|   IBIS model for TI AM261
[IBIS Ver]   5.1
[Disclaimer]   Please be aware that in the absence of a written agreement
|   Texas Instruments(TI) assumes no liability for:
|   (1) The accuracy of the IBIS models provided to your company,
|   however, the IBIS model is compliant to industry standard
|   IQ Level 2a.  Refer to IBIS Quality Section below for
|   for full details.
|   (2) The proper functioning of these Models in your design
|   or for any resulting applications
|   (3) Infringement of patents, copyrights or intellectual
|   property rights resulting from your use of these
|   models.
|   TI provides IBIS Models as a service to our customers and
|   therefore reserves the right to limit distribution of the
|   Models.  The information is subject to change without notice.
[File Name]  zcz.ibs
[File Rev]   0.1
|   -Initial version
|   -Updated Package model
[Date]   10 October 2024
[Source]   Texas Instruments Incorporated
[Copyright]   Property of Texas Instruments Incorporated.
|   Unauthorized reproduction and/or distribution is strictly.
|   prohibited.
|   This product is protected under copyright law and trade
|   secret law as an unpublished work.
|   Created 2012,(C) Copyright 1999-2012,
|   Texas Instruments Incorporated., All Rights Reserved.
|   These commodities are under the U.S. Government
|   distribution license control. As such,they are not to be
|   re-exported without the prior approval of the U.S.
|   Department of Commerce.
[Notes]
   ADC pins are marked as NC
   USB pins are marked as NC
   Clock pins are marked as NC
   nReset pin marked as NC
|   Revision History
|   GERNERAL COMMENT: All IBIS Quality Notes below reflect latest release
|   and version of IBIS File
|   File passes ibischk6.0 with 0 errors and 35 warnings
|   Component AM261
[Component] AM261
[Manufacturer] TEXAS INSTRUMENTS
[Package Model] AM261_ZCZ
[Package]
|   typ   min   max
R_pkg   0.22926   0.10115   0.40448
L_pkg   4.031e-9   1.747e-9   8.28e-9
C_pkg   5.339e-13   3.606e-13   8.638e-13
[Pin]   Signal_name   model_name
E9   VDD   POWER
E11   VDD   POWER
F9   VDD   POWER
F11   VDD   POWER
G5   VDD   POWER
G6   VDD   POWER
G13   VDD   POWER
G14   VDD   POWER
K5   VDD   POWER
K6   VDD   POWER
K13   VDD   POWER
K14   VDD   POWER
N5   VDD   POWER
N6   VDD   POWER
N13   VDD   POWER
N14   VDD   POWER
R6   VDDA18_LDO   POWER
R8   VDDA18_LDO   POWER
R11   VDDA18_LDO   POWER
R4   VDDA18_OSC_PLL   POWER
P7   VDDA33   POWER
P9   VDDA33   POWER
P11   VDDA33   POWER
D10   VDDAR2   POWER
H3   VDDAR3   POWER
D6   VDDS18   POWER
E15   VDDS18   POWER
L4   VDDS18   POWER
N15   VDDS18   POWER
T3   VDDS18_LDO   POWER
D8   VDDS33   POWER
D12   VDDS33   POWER
H4   VDDS33   POWER
H15   VDDS33   POWER
L15   VDDS33   POWER
P4   VDDS33   POWER
R15   VDDS33   POWER
T4   VDD_TEMP   NC
J16   VNWA   POWER
N3   VPP   POWER
V15   ADC0_AIN0   NC
U15   ADC0_AIN1   NC
T14   ADC0_AIN2   NC
U14   ADC0_AIN3   NC
U13   ADC0_AIN4   NC
R14   ADC0_AIN5   NC
T11   ADC1_AIN0   NC
U11   ADC1_AIN1   NC
T12   ADC1_AIN2   NC
V12   ADC1_AIN3   NC
U12   ADC1_AIN4   NC
R12   ADC1_AIN5   NC
R10   ADC2_AIN0   NC
T10   ADC2_AIN1   NC
U10   ADC2_AIN2   NC
T9   ADC2_AIN3   NC
V9   ADC2_AIN4   NC
T8   ADC2_AIN5   NC
U16   ADC_CAL0   NC
V14   ADC_VREFHI_G0   NC
V10   ADC_VREFHI_G1   NC
V13   ADC_VREFLO_G0   NC
V11   ADC_VREFLO_G1   NC
T6   ATESTV1   NC
M2   CLKOUT0   bc1833dv40dcpbfbp18ll_rxll_ssdlv
T5   DAC_OUT   NC
T13   DAC_VREF0   NC
B2   EPWM0_A   bc1833dv40dcpbfbp18ll_rxll_ssdlh_135u
B1   EPWM0_B   bc1833dv40dcpbfbp18ll_rxll_ssdlh_135u
D3   EPWM1_A   bc1833dv40dcpbfbp18ll_rxll_ssdlh_135u
D2   EPWM1_B   bc1833dv40dcpbfbp18ll_rxll_ssdlh_135u
C2   EPWM2_A   bc1833dv40dcpbfbp18ll_rxll_ssdlh_135u
C1   EPWM2_B   bc1833dv40dcpbfbp18ll_rxll_ssdlh_135u
E2   EPWM3_A   bc1833dv40dcpbfbp18ll_rxll_ssdlh_135u
E3   EPWM3_B   bc1833dv40dcpbfbp18ll_rxll_ssdlv
D1   EPWM4_A   bc1833dv40dcpbfbp18ll_rxll_ssdlv
E4   EPWM4_B   bc1833dv40dcpbfbp18ll_rxll_ssdlv
F2   EPWM5_A   bc1833dv40dcpbfbp18ll_rxll_ssdlv
G2   EPWM5_B   bc1833dv40dcpbfbp18ll_rxll_ssdlv
E1   EPWM6_A   bc1833dv40dcpbfbp18ll_rxll_ssdlv
F3   EPWM6_B   bc1833dv40dcpbfbp18ll_rxll_ssdlv
F4   EPWM7_A   bc1833dv40dcpbfbp18ll_rxll_ssdlv
F1   EPWM7_B   bc1833dv40dcpbfbp18ll_rxll_ssdlv
G3   EPWM8_A   bc1833dv40dcpbfbp18ll_rxll_ssdlv
H2   EPWM8_B   bc1833dv40dcpbfbp18ll_rxll_ssdlv
G1   EPWM9_A   bc1833dv40dcpbfbp18ll_rxll_ssdlv
J2   EPWM9_B   bc1833dv40dcpbfbp18ll_rxll_ssdlv
B14   EQEP0_A   bc1833dv40dcpbfbp18ll_rxll_ssdlh
A14   EQEP0_B   bc1833dv40dcpbfbp18ll_rxll_ssdlh
D11   EQEP0_INDEX   bc1833dv40dcpbfbp18ll_rxll_ssdlh
C12   EQEP0_STROBE   bc1833dv40dcpbfbp18ll_rxll_ssdlh
P2   EXT_REFCLK0   bc1833dv40dcpbfbp18ll_rxll_ssdlh
G4   GPIO63   bc1833dv40dcpbfbp18ll_rxll_ssdlv
J3   GPIO64   bc1833dv40dcpbfbp18ll_rxll_ssdlv
H1   GPIO65   bc1833dv40dcpbfbp18ll_rxll_ssdlv
J1   GPIO66   bc1833dv40dcpbfbp18ll_rxll_ssdlv
B12   GPIO136   bc1833dv40dcpbfbp18ll_rxll_ssdlv
A12   GPIO137   bc1833dv40dcpbfbp18ll_rxll_ssdlv
A13   I2C0_SCL   bi2c1833dvfzp18_ssdlh
B13   I2C0_SDA   bi2c1833dvfzp18_ssdlh
D7   I2C1_SCL   bc1833dv40dcpbfbp18ll_rxll_ssdlh
C8   I2C1_SDA   bc1833dv40dcpbfbp18ll_rxll_ssdlh
A9   LIN1_RXD   bc1833dv40dcpbfbp18ll_rxll_ssdlh
B9   LIN1_TXD   bc1833dv40dcpbfbp18ll_rxll_ssdlh
B8   LIN2_RXD   bc1833dv40dcpbfbp18ll_rxll_ssdlh
A8   LIN2_TXD   bc1833dv40dcpbfbp18ll_rxll_ssdlh
M1   MCAN0_RX   bc1833dv40dcpbfbp18ll_rxll_ssdlv
L1   MCAN0_TX   bc1833dv40dcpbfbp18ll_rxll_ssdlv
L2   MCAN1_RX   bc1833dv40dcpbfbp18ll_rxll_ssdlv
K1   MCAN1_TX   bc1833dv40dcpbfbp18ll_rxll_ssdlv
M17   MDIO0_MDC   bc1833dv40dcpbfbp18ll_rxll_ssdlv_135u
N16   MDIO0_MDIO   bc1833dv40dcpbfbp18ll_rxll_ssdlv_135u
A5   MMC0_CD   bc1833dv40dcpbfbp18ll_rxll_ssdlh_135u
B6   MMC0_CLK   bc1833dv40dcpbfbp18ll_rxll_ssdlh_135u
A4   MMC0_CMD   bc1833dv40dcpbfbp18ll_rxll_ssdlh_135u
B5   MMC0_D0   bc1833dv40dcpbfbp18ll_rxll_ssdlh_135u
B4   MMC0_D1   bc1833dv40dcpbfbp18ll_rxll_ssdlh_135u
A3   MMC0_D2   bc1833dv40dcpbfbp18ll_rxll_ssdlh_135u
A2   MMC0_D3   bc1833dv40dcpbfbp18ll_rxll_ssdlh_135u
C6   MMC0_WP   bc1833dv40dcpbfbp18ll_rxll_ssdlh_135u
R2   PORZ   ihhv1833dvhyp18ll_ssdhv
L18   PR0_MDIO0_MDC   bc1833dv40dcpbfbp18ll_rxll_ssdlv_135u
L17   PR0_MDIO0_MDIO   bc1833dv40dcpbfbp18ll_rxll_ssdlv_135u
K17   PR0_PRU0_GPO0   bc1833dv40dcpbfbp18ll_rxll_ssdlv_135u
K18   PR0_PRU0_GPO1   bc1833dv40dcpbfbp18ll_rxll_ssdlv_135u
J18   PR0_PRU0_GPO2   bc1833dv40dcpbfbp18ll_rxll_ssdlv_135u
J17   PR0_PRU0_GPO3   bc1833dv40dcpbfbp18ll_rxll_ssdlv_135u
K16   PR0_PRU0_GPO4   bc1833dv40dcpbfbp18ll_rxll_ssdlv_135u
G17   PR0_PRU0_GPO5   bc1833dv40dcpbfbp18ll_rxll_ssdlv_135u
K15   PR0_PRU0_GPO6   bc1833dv40dcpbfbp18ll_rxll_ssdlv_135u
G15   PR0_PRU0_GPO8   bc1833dv40dcpbfbp18ll_rxll_ssdlv_135u
F17   PR0_PRU0_GPO9   bc1833dv40dcpbfbp18ll_rxll_ssdlv_135u
G18   PR0_PRU0_GPO10   bc1833dv40dcpbfbp18ll_rxll_ssdlv_135u
M16   PR0_PRU0_GPO11   bc1833dv40dcpbfbp18ll_rxll_ssdlv_135u
M15   PR0_PRU0_GPO12   bc1833dv40dcpbfbp18ll_rxll_ssdlv_135u
H17   PR0_PRU0_GPO13   bc1833dv40dcpbfbp18ll_rxll_ssdlv_135u
H16   PR0_PRU0_GPO14   bc1833dv40dcpbfbp18ll_rxll_ssdlv_135u
L16   PR0_PRU0_GPO15   bc1833dv40dcpbfbp18ll_rxll_ssdlv_135u
H18   PR0_PRU0_GPO16   bc1833dv40dcpbfbp18ll_rxll_ssdlv_135u
F18   PR0_PRU1_GPO0   bc1833dv40dcpbfbp18ll_rxll_ssdlv_135u
G16   PR0_PRU1_GPO1   bc1833dv40dcpbfbp18ll_rxll_ssdlv_135u
E17   PR0_PRU1_GPO2   bc1833dv40dcpbfbp18ll_rxll_ssdlv_135u
E18   PR0_PRU1_GPO3   bc1833dv40dcpbfbp18ll_rxll_ssdlv_135u
F16   PR0_PRU1_GPO4   bc1833dv40dcpbfbp18ll_rxll_ssdlv_135u
F15   PR0_PRU1_GPO5   bc1833dv40dcpbfbp18ll_rxll_ssdlv_135u
E16   PR0_PRU1_GPO6   bc1833dv40dcpbfbp18ll_rxll_ssdlv_135u
D18   PR0_PRU1_GPO8   bc1833dv40dcpbfbp18ll_rxll_ssdlv_135u
C18   PR0_PRU1_GPO9   bc1833dv40dcpbfbp18ll_rxll_ssdlv_135u
D17   PR0_PRU1_GPO10   bc1833dv40dcpbfbp18ll_rxll_ssdlv_135u
B18   PR0_PRU1_GPO11   bc1833dv40dcpbfbp18ll_rxll_ssdlv_135u
B17   PR0_PRU1_GPO12   bc1833dv40dcpbfbp18ll_rxll_ssdlv_135u
D16   PR0_PRU1_GPO13   bc1833dv40dcpbfbp18ll_rxll_ssdlv_135u
C17   PR0_PRU1_GPO14   bc1833dv40dcpbfbp18ll_rxll_ssdlv_135u
A17   PR0_PRU1_GPO15   bc1833dv40dcpbfbp18ll_rxll_ssdlv_135u
C16   PR0_PRU1_GPO16   bc1833dv40dcpbfbp18ll_rxll_ssdlv_135u
C15   PR0_PRU1_GPO18   bc1833dv40dcpbfbp18ll_rxll_ssdlv_135u
D15   PR0_PRU1_GPO19   bc1833dv40dcpbfbp18ll_rxll_ssdlh
K2   PR1_PRU0_GPO0   bc1833dv40dcpbfbp18ll_rxll_ssdlv
J4   PR1_PRU0_GPO1   bc1833dv40dcpbfbp18ll_rxll_ssdlv
K4   PR1_PRU0_GPO2   bc1833dv40dcpbfbp18ll_rxll_ssdlv
K3   PR1_PRU0_GPO9   bc1833dv40dcpbfbp18ll_rxll_ssdlv
V17   PR1_PRU1_GPO0   bc1833dv40dcpbfbp18ll_rxll_ssdlh
T16   PR1_PRU1_GPO1   bc1833dv40dcpbfbp18ll_rxll_ssdlh
P15   PR1_PRU1_GPO2   bc1833dv40dcpbfbp18ll_rxll_ssdlh
R16   PR1_PRU1_GPO9   bc1833dv40dcpbfbp18ll_rxll_ssdlh
N2   QSPI0_CLK   bc1833dv40dcpbfbp18ll_rxll_ssdlv
P1   QSPI0_CSN0   bc1833dv40dcpbfbp18ll_rxll_ssdlv
R3   QSPI0_CSN1   bc1833dv40dcpbfbp18ll_rxll_ssdlv
N1   QSPI0_D0   bc1833dv40dcpbfbp18ll_ssdlv
N4   QSPI0_D1   bc1833dv40dcpbfbp18ll_ssdlv
M4   QSPI0_D2   bc1833dv40dcpbfbp18ll_rxll_ssdlv
P3   QSPI0_D3   bc1833dv40dcpbfbp18ll_rxll_ssdlv
U17   RGMII1_RD0   bc1833dv40dcpbfbp18ll_rxll_ssdlh
T17   RGMII1_RD1   bc1833dv40dcpbfbp18ll_rxll_ssdlh
U18   RGMII1_RD2   bc1833dv40dcpbfbp18ll_rxll_ssdlh
T18   RGMII1_RD3   bc1833dv40dcpbfbp18ll_rxll_ssdlv_135u
R17   RGMII1_RXC   bc1833dv40dcpbfbp18ll_rxll_ssdlv_135u
R18   RGMII1_RX_CTL   bc1833dv40dcpbfbp18ll_rxll_ssdlv_135u
P16   RGMII1_TD0   bc1833dv40dcpbfbp18ll_rxll_ssdlv_135u
P17   RGMII1_TD1   bc1833dv40dcpbfbp18ll_rxll_ssdlv_135u
P18   RGMII1_TD2   bc1833dv40dcpbfbp18ll_rxll_ssdlv_135u
N17   RGMII1_TD3   bc1833dv40dcpbfbp18ll_rxll_ssdlv_135u
N18   RGMII1_TXC   bc1833dv40dcpbfbp18ll_rxll_ssdlv_135u
M18   RGMII1_TX_CTL   bc1833dv40dcpbfbp18ll_rxll_ssdlv_135u
D4   SAFETY_ERRORN   bc1833dv40dcpbfbp18ll_ssdlh_135u
B16   SDFM0_CLK0   bc1833dv40dcpbfbp18ll_rxll_ssdlh
A16   SDFM0_CLK1   bc1833dv40dcpbfbp18ll_rxll_ssdlh
B15   SDFM0_CLK2   bc1833dv40dcpbfbp18ll_rxll_ssdlh
A15   SDFM0_CLK3   bc1833dv40dcpbfbp18ll_rxll_ssdlh
D14   SDFM0_D0   bc1833dv40dcpbfbp18ll_rxll_ssdlh
D13   SDFM0_D1   bc1833dv40dcpbfbp18ll_rxll_ssdlh
C13   SDFM0_D2   bc1833dv40dcpbfbp18ll_rxll_ssdlh
C14   SDFM0_D3   bc1833dv40dcpbfbp18ll_rxll_ssdlh
A11   SPI0_CLK   bc1833dv40dcpbfbp18ll_ssdlh
C11   SPI0_CS0   bc1833dv40dcpbfbp18ll_rxll_ssdlh
C10   SPI0_D0   bc1833dv40dcpbfbp18ll_ssdlh
B11   SPI0_D1   bc1833dv40dcpbfbp18ll_rxll_ssdlh
A10   SPI1_CLK   bc1833dv40dcpbfbp18ll_rxll_ssdlh
C9   SPI1_CS0   bc1833dv40dcpbfbp18ll_rxll_ssdlh
B10   SPI1_D0   bc1833dv40dcpbfbp18ll_rxll_ssdlh
D9   SPI1_D1   bc1833dv40dcpbfbp18ll_rxll_ssdlh
B3   TCK   iq1833dvtckpbfbp18ll_ssdhh_135u
C5   TDI   bc1833dv40dcpbfbp18ll_ssdlh_135u
C4   TDO   bc1833dv40dcpbfbp18ll_ssdlh_135u
U1   TEMPCAL   NC
D5   TMS   bc1833dv40dcpbfbp18ll_ssdlh_135u
B7   UART0_CTSN   bc1833dv40dcpbfbp18ll_rxll_ssdlh
C7   UART0_RTSN   bc1833dv40dcpbfbp18ll_rxll_ssdlh
A7   UART0_RXD   bc1833dv40dcpbfbp18ll_rxll_ssdlh
A6   UART0_TXD   bc1833dv40dcpbfbp18ll_rxll_ssdlh
L3   UART1_RXD   bc1833dv40dcpbfbp18ll_rxll_ssdlv
M3   UART1_TXD   bc1833dv40dcpbfbp18ll_rxll_ssdlv
U3   USB0_DM   NC
V2   USB0_DP   NC
U2   VSYS_MON   NC
C3   WARMRSTN   bc1833dv40dcpbfbp18ll_od_fs_cmphdl_ssdlv
T1   XTAL_XI   NC
R1   XTAL_XO   NC
A1   VSS   GND
A18   VSS   GND
E5   VSS   GND
E6   VSS   GND
E7   VSS   GND
E8   VSS   GND
E10   VSS   GND
E12   VSS   GND
E13   VSS   GND
E14   VSS   GND
F5   VSS   GND
F6   VSS   GND
F7   VSS   GND
F8   VSS   GND
F10   VSS   GND
F12   VSS   GND
F13   VSS   GND
F14   VSS   GND
G7   VSS   GND
G8   VSS   GND
G9   VSS   GND
G10   VSS   GND
G11   VSS   GND
G12   VSS   GND
H5   VSS   GND
H6   VSS   GND
H7   VSS   GND
H8   VSS   GND
H9   VSS   GND
H10   VSS   GND
H11   VSS   GND
H12   VSS   GND
H13   VSS   GND
H14   VSS   GND
J5   VSS   GND
J6   VSS   GND
J7   VSS   GND
J8   VSS   GND
J9   VSS   GND
J10   VSS   GND
J11   VSS   GND
J12   VSS   GND
J13   VSS   GND
J14   VSS   GND
K7   VSS   GND
K8   VSS   GND
K9   VSS   GND
K10   VSS   GND
K11   VSS   GND
K12   VSS   GND
L5   VSS   GND
L6   VSS   GND
L7   VSS   GND
L8   VSS   GND
L9   VSS   GND
L10   VSS   GND
L11   VSS   GND
L12   VSS   GND
L13   VSS   GND
L14   VSS   GND
M5   VSS   GND
M6   VSS   GND
M7   VSS   GND
M8   VSS   GND
M9   VSS   GND
M10   VSS   GND
M11   VSS   GND
M12   VSS   GND
M13   VSS   GND
M14   VSS   GND
N7   VSS   GND
N8   VSS   GND
N9   VSS   GND
N10   VSS   GND
N11   VSS   GND
N12   VSS   GND
P5   VSS   GND
P13   VSS   GND
P14   VSS   GND
T2   VSS   GND
V18   VSS   GND
P6   VSSA   GND
P8   VSSA   GND
P10   VSSA   GND
P12   VSSA   GND
R5   VSSA   GND
R13   VSSA   GND
V1   VSSA   GND
V16   VSSA   GND
|   BC1833DV40DCPBFBP18LL_SSDLH
[Model Selector] bc1833dv40dcpbfbp18ll_ssdlh
|SC1 IS A SLEW RATE CONTROL PIN
|5% SUPPLY VARIATION MODES WITH 1.8V NOM SUPPLY
BC40D_H_PUPDOFF_5P_SC1_1P8  Cell operated at 1.8(nom)
|BC40D_H_PUPDOFF_5P_SC1_1P8; BUFFER WITH WEAK PULUP/PULLDOWN OFF AT 5% SUPPLY
|VARIATION WITH SC1=1 MEANING SLOW MODE OF OPERATION
BC40D_H_PD_ON_5P_!SC1_1P8  Cell operated at 1.8(nom)
|BC40D_H_PD_ON_5P_!SC1_1P8; BUFFER WITH WEAK_PULLDOWN_ON AT 5% SUPPLY
|VARIATION WITH SC1=0 MEANING FAST MODE OF OPERATION
BC40D_H_PD_ON_5P_SC1_1P8  Cell operated at 1.8(nom)
|BC40D_H_PD_ON_5P_SC1_1P8; BUFFER WITH WEAK_PULLDOWN_ON AT 5% SUPPLY
|VARIATION WITH SC1=1 MEANING SLOW MODE OF OPERATION
BC40D_H_PU_ON_5P_!SC1_1P8  Cell operated at 1.8(nom)
|BC40D_H_PU_ON_5P_!SC1_1P8; BUFFER WITH WEAK_PULLUP_ON AT 5% SUPPLY
|VARIATION WITH SC1=0 MEANING FAST MODE OF OPERATION
BC40D_H_PUPDOFF_5P_!SC1_1P8  Cell operated at 1.8(nom)
|BC40D_H_PUPDOFF_5P_!SC1_1P8; BUFFER WITH WEAK PULUP/PULLDOWN OFF AT 5% SUPPLY
|VARIATION WITH SC1=0 MEANING FAST MODE OF OPERATION
BC40D_H_PU_ON_5P_SC1_1P8  Cell operated at 1.8(nom)
|BC40D_H_PU_ON_5P_SC1_1P8; BUFFER WITH WEAK_PULLUP_ON AT 5% SUPPLY
|VARIATION WITH SC1=1 MEANING SLOW MODE OF OPERATION
|5% SUPPLY VARIATION MODES WITH 3.3V NOM SUPPLY
BC40D_H_PUPDOFF_5P_SC1_3P3  Cell operated at 3.3(nom)
|BC40D_H_PUPDOFF_5P_SC1_3P3; BUFFER WITH WEAK PULUP/PULLDOWN OFF AT 5% SUPPLY
|VARIATION WITH SC1=1 MEANING SLOW MODE OF OPERATION
BC40D_H_PD_ON_5P_!SC1_3P3  Cell operated at 3.3(nom)
|BC40D_H_PD_ON_5P_!SC1_3P3; BUFFER WITH WEAK_PULLDOWN_ON AT 5% SUPPLY
|VARIATION WITH SC1=0 MEANING FAST MODE OF OPERATION
BC40D_H_PD_ON_5P_SC1_3P3  Cell operated at 3.3(nom)
|BC40D_H_PD_ON_5P_SC1_3P3; BUFFER WITH WEAK_PULLDOWN_ON AT 5% SUPPLY
|VARIATION WITH SC1=1 MEANING SLOW MODE OF OPERATION
BC40D_H_PU_ON_5P_!SC1_3P3  Cell operated at 3.3(nom)
|BC40D_H_PU_ON_5P_!SC1_3P3; BUFFER WITH WEAK_PULLUP_ON AT 5% SUPPLY
|VARIATION WITH SC1=0 MEANING FAST MODE OF OPERATION
BC40D_H_PUPDOFF_5P_!SC1_3P3  Cell operated at 3.3(nom)
|BC40D_H_PUPDOFF_5P_!SC1_3P3; BUFFER WITH WEAK PULUP/PULLDOWN OFF AT 5% SUPPLY
|VARIATION WITH SC1=0 MEANING FAST MODE OF OPERATION
BC40D_H_PU_ON_5P_SC1_3P3  Cell operated at 3.3(nom)
|BC40D_H_PU_ON_5P_SC1_3P3; BUFFER WITH WEAK_PULLUP_ON AT 5% SUPPLY
|VARIATION WITH SC1=1 MEANING SLOW MODE OF OPERATION
| 10% SUPPLY VARIATION MODES WITH 1.8V NOM SUPPLY
BC40D_H_PUPDOFF_10P_SC1_1P8  Cell operated at 1.8(nom)
|BC40D_H_PUPDOFF_10P_SC1_1P8; BUFFER WITH WEAK PULUP/PULLDOWN OFF AT 10% SUPPLY
|VARIATION WITH SC1=1 MEANING SLOW MODE OF OPERATION
BC40D_H_PD_ON_10P_!SC1_1P8  Cell operated at 1.8(nom)
|BC40D_H_PD_ON_10P_!SC1_1P8; BUFFER WITH WEAK_PULLDOWN_ON AT 10% SUPPLY
|VARIATION WITH SC1=0 MEANING FAST MODE OF OPERATION
BC40D_H_PD_ON_10P_SC1_1P8  Cell operated at 1.8(nom)
|BC40D_H_PD_ON_10P_SC1_1P8; BUFFER WITH WEAK_PULLDOWN_ON AT 10% SUPPLY
|VARIATION WITH SC1=1 MEANING SLOW MODE OF OPERATION
BC40D_H_PU_ON_10P_!SC1_1P8  Cell operated at 1.8(nom)
|BC40D_H_PU_ON_10P_!SC1_1P8; BUFFER WITH WEAK_PULLUP_ON AT 10% SUPPLY
|VARIATION WITH SC1=0 MEANING FAST MODE OF OPERATION
BC40D_H_PUPDOFF_10P_!SC1_1P8  Cell operated at 1.8(nom)
|BC40D_H_PUPDOFF_10P_!SC1_1P8; BUFFER WITH WEAK PULUP/PULLDOWN OFF AT 10% SUPPLY
|VARIATION WITH SC1=0 MEANING FAST MODE OF OPERATION
BC40D_H_PU_ON_10P_SC1_1P8  Cell operated at 1.8(nom)
|BC40D_H_PU_ON_10P_SC1_1P8; BUFFER WITH WEAK_PULLUP_ON AT 10% SUPPLY
|VARIATION WITH SC1=1 MEANING SLOW MODE OF OPERATION
| 10% SUPPLY VARIATION MODES WITH 3.3V NOM SUPPLY
BC40D_H_PUPDOFF_10P_SC1_3P3  Cell operated at 3.3(nom)
|BC40D_H_PUPDOFF_10P_SC1_3P3; BUFFER WITH WEAK PULUP/PULLDOWN OFF AT 10% SUPPLY
|VARIATION WITH SC1=1 MEANING SLOW MODE OF OPERATION
BC40D_H_PD_ON_10P_!SC1_3P3  Cell operated at 3.3(nom)
|BC40D_H_PD_ON_10P_!SC1_3P3; BUFFER WITH WEAK_PULLDOWN_ON 10% SUPPLY
|VARIATION WITH SC1=0 MEANING FAST MODE OF OPERATION
BC40D_H_PD_ON_10P_SC1_3P3  Cell operated at 3.3(nom)
|BC40D_H_PD_ON_10P_SC1_3P3; BUFFER WITH WEAK_PULLDOWN_ON AT 10% SUPPLY
|VARIATION WITH SC1=1 MEANING SLOW MODE OF OPERATION
BC40D_H_PU_ON_10P_!SC1_3P3  Cell operated at 3.3(nom)
|BC40D_H_PU_ON_10P_!SC1_3P3; BUFFER WITH WEAK_PULLUP_ON AT 10% SUPPLY
|VARIATION WITH SC1=0 MEANING FAST MODE OF OPERATION
BC40D_H_PUPDOFF_10P_!SC1_3P3  Cell operated at 3.3(nom)
|BC40D_H_PUPDOFF_10P_!SC1_3P3; BUFFER WITH WEAK PULUP/PULLDOWN OFF AT 10% SUPPLY
|VARIATION WITH SC1=0 MEANING FAST MODE OF OPERATION
BC40D_H_PU_ON_10P_SC1_3P3  Cell operated at 3.3(nom)
|BC40D_H_PU_ON_10P_SC1_3P3; BUFFER WITH WEAK_PULLUP_ON AT 10% SUPPLY
|VARIATION WITH SC1=1 MEANING SLOW MODE OF OPERATION
|   BC1833DV40DCPBFBP18LL_SSDLV
[Model Selector] bc1833dv40dcpbfbp18ll_ssdlv
|SC1 IS A SLEW RATE CONTROL PIN
|5% SUPPLY VARIATION MODES WITH 1.8V NOM SUPPLY
BC40D_V_PUPDOFF_5P_SC1_1P8  Cell operated at 1.8(nom)
|BC40D_V_PUPDOFF_5P_SC1_1P8; BUFFER WITH WEAK PULUP/PULLDOWN OFF AT 5% SUPPLY
|VARIATION WITH SC1=1 MEANING SLOW MODE OF OPERATION
BC40D_V_PD_ON_5P_!SC1_1P8  Cell operated at 1.8(nom)
|BC40D_V_PD_ON_5P_!SC1_1P8; BUFFER WITH WEAK_PULLDOWN_ON AT 5% SUPPLY
|VARIATION WITH SC1=0 MEANING FAST MODE OF OPERATION
BC40D_V_PD_ON_5P_SC1_1P8  Cell operated at 1.8(nom)
|BC40D_V_PD_ON_5P_SC1_1P8; BUFFER WITH WEAK_PULLDOWN_ON AT 5% SUPPLY
|VARIATION WITH SC1=1 MEANING SLOW MODE OF OPERATION
BC40D_V_PU_ON_5P_!SC1_1P8  Cell operated at 1.8(nom)
|BC40D_V_PU_ON_5P_!SC1_1P8; BUFFER WITH WEAK_PULLUP_ON AT 5% SUPPLY
|VARIATION WITH SC1=0 MEANING FAST MODE OF OPERATION
BC40D_V_PUPDOFF_5P_!SC1_1P8  Cell operated at 1.8(nom)
|BC40D_V_PUPDOFF_5P_!SC1_1P8; BUFFER WITH WEAK PULUP/PULLDOWN OFF AT 5% SUPPLY
|VARIATION WITH SC1=0 MEANING FAST MODE OF OPERATION
BC40D_V_PU_ON_5P_SC1_1P8  Cell operated at 1.8(nom)
|BC40D_V_PU_ON_5P_SC1_1P8; BUFFER WITH WEAK_PULLUP_ON AT 5% SUPPLY
|VARIATION WITH SC1=1 MEANING SLOW MODE OF OPERATION
|5% SUPPLY VARIATION MODES WITH 3.3V NOM SUPPLY
BC40D_V_PUPDOFF_5P_SC1_3P3  Cell operated at 3.3(nom)
|BC40D_V_PUPDOFF_5P_SC1_3P3; BUFFER WITH WEAK PULUP/PULLDOWN OFF AT 5% SUPPLY
|VARIATION WITH SC1=1 MEANING SLOW MODE OF OPERATION
BC40D_V_PD_ON_5P_!SC1_3P3  Cell operated at 3.3(nom)
|BC40D_V_PD_ON_5P_!SC1_3P3; BUFFER WITH WEAK_PULLDOWN_ON AT 5% SUPPLY
|VARIATION WITH SC1=0 MEANING FAST MODE OF OPERATION
BC40D_V_PD_ON_5P_SC1_3P3  Cell operated at 3.3(nom)
|BC40D_V_PD_ON_5P_SC1_3P3; BUFFER WITH WEAK_PULLDOWN_ON AT 5% SUPPLY
|VARIATION WITH SC1=1 MEANING SLOW MODE OF OPERATION
BC40D_V_PU_ON_5P_!SC1_3P3  Cell operated at 3.3(nom)
|BC40D_V_PU_ON_5P_!SC1_3P3; BUFFER WITH WEAK_PULLUP_ON AT 5% SUPPLY
|VARIATION WITH SC1=0 MEANING FAST MODE OF OPERATION
BC40D_V_PUPDOFF_5P_!SC1_3P3  Cell operated at 3.3(nom)
|BC40D_V_PUPDOFF_5P_!SC1_3P3; BUFFER WITH WEAK PULUP/PULLDOWN OFF AT 5% SUPPLY
|VARIATION WITH SC1=0 MEANING FAST MODE OF OPERATION
BC40D_V_PU_ON_5P_SC1_3P3  Cell operated at 3.3(nom)
|BC40D_V_PU_ON_5P_SC1_3P3; BUFFER WITH WEAK_PULLUP_ON AT 5% SUPPLY
|VARIATION WITH SC1=1 MEANING SLOW MODE OF OPERATION
| 10% SUPPLY VARIATION MODES WITH 1.8V NOM SUPPLY
BC40D_V_PUPDOFF_10P_SC1_1P8  Cell operated at 1.8(nom)
|BC40D_V_PUPDOFF_10P_SC1_1P8; BUFFER WITH WEAK PULUP/PULLDOWN OFF AT 10% SUPPLY
|VARIATION WITH SC1=1 MEANING SLOW MODE OF OPERATION
BC40D_V_PD_ON_10P_!SC1_1P8  Cell operated at 1.8(nom)
|BC40D_V_PD_ON_10P_!SC1_1P8; BUFFER WITH WEAK_PULLDOWN_ON AT 10% SUPPLY
|VARIATION WITH SC1=0 MEANING FAST MODE OF OPERATION
BC40D_V_PD_ON_10P_SC1_1P8  Cell operated at 1.8(nom)
|BC40D_V_PD_ON_10P_SC1_1P8; BUFFER WITH WEAK_PULLDOWN_ON AT 10% SUPPLY
|VARIATION WITH SC1=1 MEANING SLOW MODE OF OPERATION
BC40D_V_PU_ON_10P_!SC1_1P8  Cell operated at 1.8(nom)
|BC40D_V_PU_ON_10P_!SC1_1P8; BUFFER WITH WEAK_PULLUP_ON AT 10% SUPPLY
|VARIATION WITH SC1=0 MEANING FAST MODE OF OPERATION
BC40D_V_PUPDOFF_10P_!SC1_1P8  Cell operated at 1.8(nom)
|BC40D_V_PUPDOFF_10P_!SC1_1P8; BUFFER WITH WEAK PULUP/PULLDOWN OFF AT 10% SUPPLY
|VARIATION WITH SC1=0 MEANING FAST MODE OF OPERATION
BC40D_V_PU_ON_10P_SC1_1P8  Cell operated at 1.8(nom)
|BC40D_V_PU_ON_10P_SC1_1P8; BUFFER WITH WEAK_PULLUP_ON AT 10% SUPPLY
|VARIATION WITH SC1=1 MEANING SLOW MODE OF OPERATION
| 10% SUPPLY VARIATION MODES WITH 3.3V NOM SUPPLY
BC40D_V_PUPDOFF_10P_SC1_3P3  Cell operated at 3.3(nom)
|BC40D_V_PUPDOFF_10P_SC1_3P3; BUFFER WITH WEAK PULUP/PULLDOWN OFF AT 10% SUPPLY
|VARIATION WITH SC1=1 MEANING SLOW MODE OF OPERATION
BC40D_V_PD_ON_10P_!SC1_3P3  Cell operated at 3.3(nom)
|BC40D_V_PD_ON_10P_!SC1_3P3; BUFFER WITH WEAK_PULLDOWN_ON 10% SUPPLY
|VARIATION WITH SC1=0 MEANING FAST MODE OF OPERATION
BC40D_V_PD_ON_10P_SC1_3P3  Cell operated at 3.3(nom)
|BC40D_V_PD_ON_10P_SC1_3P3; BUFFER WITH WEAK_PULLDOWN_ON AT 10% SUPPLY
|VARIATION WITH SC1=1 MEANING SLOW MODE OF OPERATION
BC40D_V_PU_ON_10P_!SC1_3P3  Cell operated at 3.3(nom)
|BC40D_V_PU_ON_10P_!SC1_3P3; BUFFER WITH WEAK_PULLUP_ON AT 10% SUPPLY
|VARIATION WITH SC1=0 MEANING FAST MODE OF OPERATION
BC40D_V_PUPDOFF_10P_!SC1_3P3  Cell operated at 3.3(nom)
|BC40D_V_PUPDOFF_10P_!SC1_3P3; BUFFER WITH WEAK PULUP/PULLDOWN OFF AT 10% SUPPLY
|VARIATION WITH SC1=0 MEANING FAST MODE OF OPERATION
BC40D_V_PU_ON_10P_SC1_3P3  Cell operated at 3.3(nom)
|BC40D_V_PU_ON_10P_SC1_3P3; BUFFER WITH WEAK_PULLUP_ON AT 10% SUPPLY
|VARIATION WITH SC1=1 MEANING SLOW MODE OF OPERATION
|   BI2C1833DVFZP18_SSDLH
[Model Selector] bi2c1833dvfzp18_ssdlh
BI2C1833_NORAML_5P_1P8  Cell operated at 1.8(nom)
|BI2C1833_NORAML_5P_1P8; I2C MODE AT 1.8V WITH 5% SUPPLY VARIATION
BI2C1833_NORAML_5P_3P3  Cell operated at 3.3(nom)
|BI2C1833_NORAML_5P_3P3; I2C MODE AT 3.3V WITH 5% SUPPLY VARIATION
BI2C1833_NORAML_10P_1P8  Cell operated at 1.8(nom)
|BI2C1833_NORAML_10P_1P8; I2C MODE AT 1.8V WITH 10% SUPPLY VARIATION
BI2C1833_NORAML_10P_3P3  Cell operated at 3.3(nom)
|BI2C1833_NORAML_10P_3P3; I2C MODE AT 3.3V WITH 10% SUPPLY VARIATION
|   IHHV1833DVHYP18LL_SSDHV
[Model Selector] ihhv1833dvhyp18ll_ssdhv
IHHV_NORAML_5P_1P8  Cell operated at 1.8(nom)
|IHHV_NORAML_5P_1P8; NORMAL MODE AT 1.8V WITH 5% SUPPLY VARIATION
IHHV_NORAML_5P_3P3  Cell operated at 3.3(nom)
|IHHV_NORAML_5P_3P3; NORMAL MODE AT 3.3V WITH 5% SUPPLY VARIATION
IHHV_NORAML_10P_1P8  Cell operated at 1.8(nom)
|IHHV_NORAML_10P_1P8; NORMAL MODE AT 1.8V WITH 10% SUPPLY VARIATION
IHHV_NORAML_10P_3P3  Cell operated at 3.3(nom)
|IHHV_NORAML_10P_3P3; NORMAL MODE AT 3.3V WITH 10% SUPPLY VARIATION
|   BC1833DV40DCPBFBP18LL_OD_FS_CMPHLDL_SSDLV
[Model Selector] bc1833dv40dcpbfbp18ll_od_fs_cmphdl_ssdlv
|SC1 IS A SLEW RATE CONTROL PIN
|5% SUPPLY VARIATION MODES WITH 1.8V NOM SUPPLY
BC40D_V_PUPDOFF_5P_SC1_1P8  Cell operated at 1.8(nom)
|BC40D_V_PUPDOFF_5P_SC1_1P8; BUFFER WITH WEAK PULUP/PULLDOWN OFF AT 5% SUPPLY
|VARIATION WITH SC1=1 MEANING SLOW MODE OF OPERATION
BC40D_V_PD_ON_5P_!SC1_1P8  Cell operated at 1.8(nom)
|BC40D_V_PD_ON_5P_!SC1_1P8; BUFFER WITH WEAK_PULLDOWN_ON AT 5% SUPPLY
|VARIATION WITH SC1=0 MEANING FAST MODE OF OPERATION
BC40D_V_PD_ON_5P_SC1_1P8  Cell operated at 1.8(nom)
|BC40D_V_PD_ON_5P_SC1_1P8; BUFFER WITH WEAK_PULLDOWN_ON AT 5% SUPPLY
|VARIATION WITH SC1=1 MEANING SLOW MODE OF OPERATION
BC40D_V_PU_ON_5P_!SC1_1P8  Cell operated at 1.8(nom)
|BC40D_V_PU_ON_5P_!SC1_1P8; BUFFER WITH WEAK_PULLUP_ON AT 5% SUPPLY
|VARIATION WITH SC1=0 MEANING FAST MODE OF OPERATION
BC40D_V_PUPDOFF_5P_!SC1_1P8  Cell operated at 1.8(nom)
|BC40D_V_PUPDOFF_5P_!SC1_1P8; BUFFER WITH WEAK PULUP/PULLDOWN OFF AT 5% SUPPLY
|VARIATION WITH SC1=0 MEANING FAST MODE OF OPERATION
BC40D_V_PU_ON_5P_SC1_1P8  Cell operated at 1.8(nom)
|BC40D_V_PU_ON_5P_SC1_1P8; BUFFER WITH WEAK_PULLUP_ON AT 5% SUPPLY
|VARIATION WITH SC1=1 MEANING SLOW MODE OF OPERATION
|5% SUPPLY VARIATION MODES WITH 3.3V NOM SUPPLY
BC40D_V_PUPDOFF_5P_SC1_3P3  Cell operated at 3.3(nom)
|BC40D_V_PUPDOFF_5P_SC1_3P3; BUFFER WITH WEAK PULUP/PULLDOWN OFF AT 5% SUPPLY
|VARIATION WITH SC1=1 MEANING SLOW MODE OF OPERATION
BC40D_V_PD_ON_5P_!SC1_3P3  Cell operated at 3.3(nom)
|BC40D_V_PD_ON_5P_!SC1_3P3; BUFFER WITH WEAK_PULLDOWN_ON AT 5% SUPPLY
|VARIATION WITH SC1=0 MEANING FAST MODE OF OPERATION
BC40D_V_PD_ON_5P_SC1_3P3  Cell operated at 3.3(nom)
|BC40D_V_PD_ON_5P_SC1_3P3; BUFFER WITH WEAK_PULLDOWN_ON AT 5% SUPPLY
|VARIATION WITH SC1=1 MEANING SLOW MODE OF OPERATION
BC40D_V_PU_ON_5P_!SC1_3P3  Cell operated at 3.3(nom)
|BC40D_V_PU_ON_5P_!SC1_3P3; BUFFER WITH WEAK_PULLUP_ON AT 5% SUPPLY
|VARIATION WITH SC1=0 MEANING FAST MODE OF OPERATION
BC40D_V_PUPDOFF_5P_!SC1_3P3  Cell operated at 3.3(nom)
|BC40D_V_PUPDOFF_5P_!SC1_3P3; BUFFER WITH WEAK PULUP/PULLDOWN OFF AT 5% SUPPLY
|VARIATION WITH SC1=0 MEANING FAST MODE OF OPERATION
BC40D_V_PU_ON_5P_SC1_3P3  Cell operated at 3.3(nom)
|BC40D_V_PU_ON_5P_SC1_3P3; BUFFER WITH WEAK_PULLUP_ON AT 5% SUPPLY
|VARIATION WITH SC1=1 MEANING SLOW MODE OF OPERATION
| 10% SUPPLY VARIATION MODES WITH 1.8V NOM SUPPLY
BC40D_V_PUPDOFF_10P_SC1_1P8  Cell operated at 1.8(nom)
|BC40D_V_PUPDOFF_10P_SC1_1P8; BUFFER WITH WEAK PULUP/PULLDOWN OFF AT 10% SUPPLY
|VARIATION WITH SC1=1 MEANING SLOW MODE OF OPERATION
BC40D_V_PD_ON_10P_!SC1_1P8  Cell operated at 1.8(nom)
|BC40D_V_PD_ON_10P_!SC1_1P8; BUFFER WITH WEAK_PULLDOWN_ON AT 10% SUPPLY
|VARIATION WITH SC1=0 MEANING FAST MODE OF OPERATION
BC40D_V_PD_ON_10P_SC1_1P8  Cell operated at 1.8(nom)
|BC40D_V_PD_ON_10P_SC1_1P8; BUFFER WITH WEAK_PULLDOWN_ON AT 10% SUPPLY
|VARIATION WITH SC1=1 MEANING SLOW MODE OF OPERATION
BC40D_V_PU_ON_10P_!SC1_1P8  Cell operated at 1.8(nom)
|BC40D_V_PU_ON_10P_!SC1_1P8; BUFFER WITH WEAK_PULLUP_ON AT 10% SUPPLY
|VARIATION WITH SC1=0 MEANING FAST MODE OF OPERATION
BC40D_V_PUPDOFF_10P_!SC1_1P8  Cell operated at 1.8(nom)
|BC40D_V_PUPDOFF_10P_!SC1_1P8; BUFFER WITH WEAK PULUP/PULLDOWN OFF AT 10% SUPPLY
|VARIATION WITH SC1=0 MEANING FAST MODE OF OPERATION
BC40D_V_PU_ON_10P_SC1_1P8  Cell operated at 1.8(nom)
|BC40D_V_PU_ON_10P_SC1_1P8; BUFFER WITH WEAK_PULLUP_ON AT 10% SUPPLY
|VARIATION WITH SC1=1 MEANING SLOW MODE OF OPERATION
| 10% SUPPLY VARIATION MODES WITH 3.3V NOM SUPPLY
BC40D_V_PUPDOFF_10P_SC1_3P3  Cell operated at 3.3(nom)
|BC40D_V_PUPDOFF_10P_SC1_3P3; BUFFER WITH WEAK PULUP/PULLDOWN OFF AT 10% SUPPLY
|VARIATION WITH SC1=1 MEANING SLOW MODE OF OPERATION
BC40D_V_PD_ON_10P_!SC1_3P3  Cell operated at 3.3(nom)
|BC40D_V_PD_ON_10P_!SC1_3P3; BUFFER WITH WEAK_PULLDOWN_ON 10% SUPPLY
|VARIATION WITH SC1=0 MEANING FAST MODE OF OPERATION
BC40D_V_PD_ON_10P_SC1_3P3  Cell operated at 3.3(nom)
|BC40D_V_PD_ON_10P_SC1_3P3; BUFFER WITH WEAK_PULLDOWN_ON AT 10% SUPPLY
|VARIATION WITH SC1=1 MEANING SLOW MODE OF OPERATION
BC40D_V_PU_ON_10P_!SC1_3P3  Cell operated at 3.3(nom)
|BC40D_V_PU_ON_10P_!SC1_3P3; BUFFER WITH WEAK_PULLUP_ON AT 10% SUPPLY
|VARIATION WITH SC1=0 MEANING FAST MODE OF OPERATION
BC40D_V_PUPDOFF_10P_!SC1_3P3  Cell operated at 3.3(nom)
|BC40D_V_PUPDOFF_10P_!SC1_3P3; BUFFER WITH WEAK PULUP/PULLDOWN OFF AT 10% SUPPLY
|VARIATION WITH SC1=0 MEANING FAST MODE OF OPERATION
BC40D_V_PU_ON_10P_SC1_3P3  Cell operated at 3.3(nom)
|BC40D_V_PU_ON_10P_SC1_3P3; BUFFER WITH WEAK_PULLUP_ON AT 10% SUPPLY
|VARIATION WITH SC1=1 MEANING SLOW MODE OF OPERATION
|   IQ1833DVTCKPBFBP18LL_SSDHH_135U
[Model Selector] iq1833dvtckpbfbp18ll_ssdhh_135u
|5% SUPPLY VARIATION MODES WITH 1.8V NOM SUPPLY
IQ_SSDHH_PD_ON_5P_1P8  Cell operated at 1.8(nom)
|IQ_SSDHH_PD_ON_5P_1P8; BUFFER WITH WEAK_PULLDOWN_ON AT 5% SUPPLY VARIATION
IQ_SSDHH_PU_ON_5P_1P8  Cell operated at 1.8(nom)
|IQ_SSDHH_PU_ON_5P_1P8; BUFFER WITH WEAK_PULLUP_ON AT 5% SUPPLY VARIATION
IQ_SSDHH_PUPDOFF_5P_1P8  Cell operated at 1.8(nom)
|IQ_SSDHH_PUPDOFF_5P_1P8; BUFFER WITH WEAK PUPD OFF AT 5% SUPPLY VARIATION
|5% SUPPLY VARIATION MODES WITH 3.3V NOM SUPPLY
IQ_SSDHH_PD_ON_5P_3P3  Cell operated at 3.3(nom)
|IQ_SSDHH_PD_ON_5P_3P3; BUFFER WITH WEAK_PULLDOWN_ON AT 5% SUPPLY VARIATION
IQ_SSDHH_PU_ON_5P_3P3  Cell operated at 3.3(nom)
|IQ_SSDHH_PU_ON_5P_3P3; BUFFER WITH WEAK_PULLUP_ON AT 5% SUPPLY VARIATION
IQ_SSDHH_PUPDOFF_5P_3P3  Cell operated at 3.3(nom)
|IQ_SSDHH_PUPDOFF_5P_3P3; BUFFER WITH WEAK PUPD OFF AT 5% SUPPLY VARIATION
|10% SUPPLY VARIATION MODES WITH 1.8V NOM SUPPLY
IQ_SSDHH_PD_ON_10P_1P8  Cell operated at 1.8(nom)
|IQ_SSDHH_PD_ON_10P_1P8; BUFFER WITH WEAK_PULLDOWN_ON AT 10% SUPPLY VARIATION
IQ_SSDHH_PU_ON_10P_1P8  Cell operated at 1.8(nom)
|IQ_SSDHH_PU_ON_10P_1P8; BUFFER WITH WEAK_PULLUP_ON AT 10% SUPPLY VARIATION
IQ_SSDHH_PUPDOFF_10P_1P8  Cell operated at 1.8(nom)
|IQ_SSDHH_PUPDOFF_10P_1P8; BUFFER WITH WEAK PUPD OFF AT 10% SUPPLY VARIATION
|10% SUPPLY VARIATION MODES WITH 3.3V NOM SUPPLY
IQ_SSDHH_PD_ON_10P_3P3  Cell operated at 3.3(nom)
|IQ_SSDHH_PD_ON_10P_3P3; BUFFER WITH WEAK_PULLDOWN_ON  AT 10% SUPPLY VARIATION
IQ_SSDHH_PU_ON_10P_3P3  Cell operated at 3.3(nom)
|IQ_SSDHH_PU_ON_10P_3P3; BUFFER WITH WEAK_PULLUP_ON AT 10% SUPPLY VARIATION
IQ_SSDHH_PUPDOFF_10P_3P3  Cell operated at 3.3(nom)
|IQ_SSDHH_PUPDOFF_10P_3P3; BUFFER WITH WEAK PUPD OFF AT 10% SUPPLY VARIATION
|   BC1833DV40DCPBFBP18LL_RXLL_SSDLH
[Model Selector] bc1833dv40dcpbfbp18ll_rxll_ssdlh
|SC1 IS A SLEW RATE CONTROL PIN
|5% SUPPLY VARIATION MODES WITH 1.8V NOM SUPPLY
BC40D_H_PUPDOFF_5P_SC1_1P8  Cell operated at 1.8(nom)
|BC40D_H_PUPDOFF_5P_SC1_1P8; BUFFER WITH WEAK PULUP/PULLDOWN OFF AT 5% SUPPLY
|VARIATION WITH SC1=1 MEANING SLOW MODE OF OPERATION
BC40D_H_PD_ON_5P_!SC1_1P8  Cell operated at 1.8(nom)
|BC40D_H_PD_ON_5P_!SC1_1P8; BUFFER WITH WEAK_PULLDOWN_ON AT 5% SUPPLY
|VARIATION WITH SC1=0 MEANING FAST MODE OF OPERATION
BC40D_H_PD_ON_5P_SC1_1P8  Cell operated at 1.8(nom)
|BC40D_H_PD_ON_5P_SC1_1P8; BUFFER WITH WEAK_PULLDOWN_ON AT 5% SUPPLY
|VARIATION WITH SC1=1 MEANING SLOW MODE OF OPERATION
BC40D_H_PU_ON_5P_!SC1_1P8  Cell operated at 1.8(nom)
|BC40D_H_PU_ON_5P_!SC1_1P8; BUFFER WITH WEAK_PULLUP_ON AT 5% SUPPLY
|VARIATION WITH SC1=0 MEANING FAST MODE OF OPERATION
BC40D_H_PUPDOFF_5P_!SC1_1P8  Cell operated at 1.8(nom)
|BC40D_H_PUPDOFF_5P_!SC1_1P8; BUFFER WITH WEAK PULUP/PULLDOWN OFF AT 5% SUPPLY
|VARIATION WITH SC1=0 MEANING FAST MODE OF OPERATION
BC40D_H_PU_ON_5P_SC1_1P8  Cell operated at 1.8(nom)
|BC40D_H_PU_ON_5P_SC1_1P8; BUFFER WITH WEAK_PULLUP_ON AT 5% SUPPLY
|VARIATION WITH SC1=1 MEANING SLOW MODE OF OPERATION
|5% SUPPLY VARIATION MODES WITH 3.3V NOM SUPPLY
BC40D_H_PUPDOFF_5P_SC1_3P3  Cell operated at 3.3(nom)
|BC40D_H_PUPDOFF_5P_SC1_3P3; BUFFER WITH WEAK PULUP/PULLDOWN OFF AT 5% SUPPLY
|VARIATION WITH SC1=1 MEANING SLOW MODE OF OPERATION
BC40D_H_PD_ON_5P_!SC1_3P3  Cell operated at 3.3(nom)
|BC40D_H_PD_ON_5P_!SC1_3P3; BUFFER WITH WEAK_PULLDOWN_ON AT 5% SUPPLY
|VARIATION WITH SC1=0 MEANING FAST MODE OF OPERATION
BC40D_H_PD_ON_5P_SC1_3P3  Cell operated at 3.3(nom)
|BC40D_H_PD_ON_5P_SC1_3P3; BUFFER WITH WEAK_PULLDOWN_ON AT 5% SUPPLY
|VARIATION WITH SC1=1 MEANING SLOW MODE OF OPERATION
BC40D_H_PU_ON_5P_!SC1_3P3  Cell operated at 3.3(nom)
|BC40D_H_PU_ON_5P_!SC1_3P3; BUFFER WITH WEAK_PULLUP_ON AT 5% SUPPLY
|VARIATION WITH SC1=0 MEANING FAST MODE OF OPERATION
BC40D_H_PUPDOFF_5P_!SC1_3P3  Cell operated at 3.3(nom)
|BC40D_H_PUPDOFF_5P_!SC1_3P3; BUFFER WITH WEAK PULUP/PULLDOWN OFF AT 5% SUPPLY
|VARIATION WITH SC1=0 MEANING FAST MODE OF OPERATION
BC40D_H_PU_ON_5P_SC1_3P3  Cell operated at 3.3(nom)
|BC40D_H_PU_ON_5P_SC1_3P3; BUFFER WITH WEAK_PULLUP_ON AT 5% SUPPLY
|VARIATION WITH SC1=1 MEANING SLOW MODE OF OPERATION
| 10% SUPPLY VARIATION MODES WITH 1.8V NOM SUPPLY
BC40D_H_PUPDOFF_10P_SC1_1P8  Cell operated at 1.8(nom)
|BC40D_H_PUPDOFF_10P_SC1_1P8; BUFFER WITH WEAK PULUP/PULLDOWN OFF AT 10% SUPPLY
|VARIATION WITH SC1=1 MEANING SLOW MODE OF OPERATION
BC40D_H_PD_ON_10P_!SC1_1P8  Cell operated at 1.8(nom)
|BC40D_H_PD_ON_10P_!SC1_1P8; BUFFER WITH WEAK_PULLDOWN_ON AT 10% SUPPLY
|VARIATION WITH SC1=0 MEANING FAST MODE OF OPERATION
BC40D_H_PD_ON_10P_SC1_1P8  Cell operated at 1.8(nom)
|BC40D_H_PD_ON_10P_SC1_1P8; BUFFER WITH WEAK_PULLDOWN_ON AT 10% SUPPLY
|VARIATION WITH SC1=1 MEANING SLOW MODE OF OPERATION
BC40D_H_PU_ON_10P_!SC1_1P8  Cell operated at 1.8(nom)
|BC40D_H_PU_ON_10P_!SC1_1P8; BUFFER WITH WEAK_PULLUP_ON AT 10% SUPPLY
|VARIATION WITH SC1=0 MEANING FAST MODE OF OPERATION
BC40D_H_PUPDOFF_10P_!SC1_1P8  Cell operated at 1.8(nom)
|BC40D_H_PUPDOFF_10P_!SC1_1P8; BUFFER WITH WEAK PULUP/PULLDOWN OFF AT 10% SUPPLY
|VARIATION WITH SC1=0 MEANING FAST MODE OF OPERATION
BC40D_H_PU_ON_10P_SC1_1P8  Cell operated at 1.8(nom)
|BC40D_H_PU_ON_10P_SC1_1P8; BUFFER WITH WEAK_PULLUP_ON AT 10% SUPPLY
|VARIATION WITH SC1=1 MEANING SLOW MODE OF OPERATION
| 10% SUPPLY VARIATION MODES WITH 3.3V NOM SUPPLY
BC40D_H_PUPDOFF_10P_SC1_3P3  Cell operated at 3.3(nom)
|BC40D_H_PUPDOFF_10P_SC1_3P3; BUFFER WITH WEAK PULUP/PULLDOWN OFF AT 10% SUPPLY
|VARIATION WITH SC1=1 MEANING SLOW MODE OF OPERATION
BC40D_H_PD_ON_10P_!SC1_3P3  Cell operated at 3.3(nom)
|BC40D_H_PD_ON_10P_!SC1_3P3; BUFFER WITH WEAK_PULLDOWN_ON 10% SUPPLY
|VARIATION WITH SC1=0 MEANING FAST MODE OF OPERATION
BC40D_H_PD_ON_10P_SC1_3P3  Cell operated at 3.3(nom)
|BC40D_H_PD_ON_10P_SC1_3P3; BUFFER WITH WEAK_PULLDOWN_ON AT 10% SUPPLY
|VARIATION WITH SC1=1 MEANING SLOW MODE OF OPERATION
BC40D_H_PU_ON_10P_!SC1_3P3  Cell operated at 3.3(nom)
|BC40D_H_PU_ON_10P_!SC1_3P3; BUFFER WITH WEAK_PULLUP_ON AT 10% SUPPLY
|VARIATION WITH SC1=0 MEANING FAST MODE OF OPERATION
BC40D_H_PUPDOFF_10P_!SC1_3P3  Cell operated at 3.3(nom)
|BC40D_H_PUPDOFF_10P_!SC1_3P3; BUFFER WITH WEAK PULUP/PULLDOWN OFF AT 10% SUPPLY
|VARIATION WITH SC1=0 MEANING FAST MODE OF OPERATION
BC40D_H_PU_ON_10P_SC1_3P3  Cell operated at 3.3(nom)
|BC40D_H_PU_ON_10P_SC1_3P3; BUFFER WITH WEAK_PULLUP_ON AT 10% SUPPLY
|VARIATION WITH SC1=1 MEANING SLOW MODE OF OPERATION
|   BC1833DV40DCPBFBP18LL_RXLL_SSDLV
[Model Selector] bc1833dv40dcpbfbp18ll_rxll_ssdlv
|SC1 IS A SLEW RATE CONTROL PIN
|5% SUPPLY VARIATION MODES WITH 1.8V NOM SUPPLY
BC40D_V_PUPDOFF_5P_SC1_1P8  Cell operated at 1.8(nom)
|BC40D_V_PUPDOFF_5P_SC1_1P8; BUFFER WITH WEAK PULUP/PULLDOWN OFF AT 5% SUPPLY
|VARIATION WITH SC1=1 MEANING SLOW MODE OF OPERATION
BC40D_V_PD_ON_5P_!SC1_1P8  Cell operated at 1.8(nom)
|BC40D_V_PD_ON_5P_!SC1_1P8; BUFFER WITH WEAK_PULLDOWN_ON AT 5% SUPPLY
|VARIATION WITH SC1=0 MEANING FAST MODE OF OPERATION
BC40D_V_PD_ON_5P_SC1_1P8  Cell operated at 1.8(nom)
|BC40D_V_PD_ON_5P_SC1_1P8; BUFFER WITH WEAK_PULLDOWN_ON AT 5% SUPPLY
|VARIATION WITH SC1=1 MEANING SLOW MODE OF OPERATION
BC40D_V_PU_ON_5P_!SC1_1P8  Cell operated at 1.8(nom)
|BC40D_V_PU_ON_5P_!SC1_1P8; BUFFER WITH WEAK_PULLUP_ON AT 5% SUPPLY
|VARIATION WITH SC1=0 MEANING FAST MODE OF OPERATION
BC40D_V_PUPDOFF_5P_!SC1_1P8  Cell operated at 1.8(nom)
|BC40D_V_PUPDOFF_5P_!SC1_1P8; BUFFER WITH WEAK PULUP/PULLDOWN OFF AT 5% SUPPLY
|VARIATION WITH SC1=0 MEANING FAST MODE OF OPERATION
BC40D_V_PU_ON_5P_SC1_1P8  Cell operated at 1.8(nom)
|BC40D_V_PU_ON_5P_SC1_1P8; BUFFER WITH WEAK_PULLUP_ON AT 5% SUPPLY
|VARIATION WITH SC1=1 MEANING SLOW MODE OF OPERATION
|5% SUPPLY VARIATION MODES WITH 3.3V NOM SUPPLY
BC40D_V_PUPDOFF_5P_SC1_3P3  Cell operated at 3.3(nom)
|BC40D_V_PUPDOFF_5P_SC1_3P3; BUFFER WITH WEAK PULUP/PULLDOWN OFF AT 5% SUPPLY
|VARIATION WITH SC1=1 MEANING SLOW MODE OF OPERATION
BC40D_V_PD_ON_5P_!SC1_3P3  Cell operated at 3.3(nom)
|BC40D_V_PD_ON_5P_!SC1_3P3; BUFFER WITH WEAK_PULLDOWN_ON AT 5% SUPPLY
|VARIATION WITH SC1=0 MEANING FAST MODE OF OPERATION
BC40D_V_PD_ON_5P_SC1_3P3  Cell operated at 3.3(nom)
|BC40D_V_PD_ON_5P_SC1_3P3; BUFFER WITH WEAK_PULLDOWN_ON AT 5% SUPPLY
|VARIATION WITH SC1=1 MEANING SLOW MODE OF OPERATION
BC40D_V_PU_ON_5P_!SC1_3P3  Cell operated at 3.3(nom)
|BC40D_V_PU_ON_5P_!SC1_3P3; BUFFER WITH WEAK_PULLUP_ON AT 5% SUPPLY
|VARIATION WITH SC1=0 MEANING FAST MODE OF OPERATION
BC40D_V_PUPDOFF_5P_!SC1_3P3  Cell operated at 3.3(nom)
|BC40D_V_PUPDOFF_5P_!SC1_3P3; BUFFER WITH WEAK PULUP/PULLDOWN OFF AT 5% SUPPLY
|VARIATION WITH SC1=0 MEANING FAST MODE OF OPERATION
BC40D_V_PU_ON_5P_SC1_3P3  Cell operated at 3.3(nom)
|BC40D_V_PU_ON_5P_SC1_3P3; BUFFER WITH WEAK_PULLUP_ON AT 5% SUPPLY
|VARIATION WITH SC1=1 MEANING SLOW MODE OF OPERATION
| 10% SUPPLY VARIATION MODES WITH 1.8V NOM SUPPLY
BC40D_V_PUPDOFF_10P_SC1_1P8  Cell operated at 1.8(nom)
|BC40D_V_PUPDOFF_10P_SC1_1P8; BUFFER WITH WEAK PULUP/PULLDOWN OFF AT 10% SUPPLY
|VARIATION WITH SC1=1 MEANING SLOW MODE OF OPERATION
BC40D_V_PD_ON_10P_!SC1_1P8  Cell operated at 1.8(nom)
|BC40D_V_PD_ON_10P_!SC1_1P8; BUFFER WITH WEAK_PULLDOWN_ON AT 10% SUPPLY
|VARIATION WITH SC1=0 MEANING FAST MODE OF OPERATION
BC40D_V_PD_ON_10P_SC1_1P8  Cell operated at 1.8(nom)
|BC40D_V_PD_ON_10P_SC1_1P8; BUFFER WITH WEAK_PULLDOWN_ON AT 10% SUPPLY
|VARIATION WITH SC1=1 MEANING SLOW MODE OF OPERATION
BC40D_V_PU_ON_10P_!SC1_1P8  Cell operated at 1.8(nom)
|BC40D_V_PU_ON_10P_!SC1_1P8; BUFFER WITH WEAK_PULLUP_ON AT 10% SUPPLY
|VARIATION WITH SC1=0 MEANING FAST MODE OF OPERATION
BC40D_V_PUPDOFF_10P_!SC1_1P8  Cell operated at 1.8(nom)
|BC40D_V_PUPDOFF_10P_!SC1_1P8; BUFFER WITH WEAK PULUP/PULLDOWN OFF AT 10% SUPPLY
|VARIATION WITH SC1=0 MEANING FAST MODE OF OPERATION
BC40D_V_PU_ON_10P_SC1_1P8  Cell operated at 1.8(nom)
|BC40D_V_PU_ON_10P_SC1_1P8; BUFFER WITH WEAK_PULLUP_ON AT 10% SUPPLY
|VARIATION WITH SC1=1 MEANING SLOW MODE OF OPERATION
| 10% SUPPLY VARIATION MODES WITH 3.3V NOM SUPPLY
BC40D_V_PUPDOFF_10P_SC1_3P3  Cell operated at 3.3(nom)
|BC40D_V_PUPDOFF_10P_SC1_3P3; BUFFER WITH WEAK PULUP/PULLDOWN OFF AT 10% SUPPLY
|VARIATION WITH SC1=1 MEANING SLOW MODE OF OPERATION
BC40D_V_PD_ON_10P_!SC1_3P3  Cell operated at 3.3(nom)
|BC40D_V_PD_ON_10P_!SC1_3P3; BUFFER WITH WEAK_PULLDOWN_ON 10% SUPPLY
|VARIATION WITH SC1=0 MEANING FAST MODE OF OPERATION
BC40D_V_PD_ON_10P_SC1_3P3  Cell operated at 3.3(nom)
|BC40D_V_PD_ON_10P_SC1_3P3; BUFFER WITH WEAK_PULLDOWN_ON AT 10% SUPPLY
|VARIATION WITH SC1=1 MEANING SLOW MODE OF OPERATION
BC40D_V_PU_ON_10P_!SC1_3P3  Cell operated at 3.3(nom)
|BC40D_V_PU_ON_10P_!SC1_3P3; BUFFER WITH WEAK_PULLUP_ON AT 10% SUPPLY
|VARIATION WITH SC1=0 MEANING FAST MODE OF OPERATION
BC40D_V_PUPDOFF_10P_!SC1_3P3  Cell operated at 3.3(nom)
|BC40D_V_PUPDOFF_10P_!SC1_3P3; BUFFER WITH WEAK PULUP/PULLDOWN OFF AT 10% SUPPLY
|VARIATION WITH SC1=0 MEANING FAST MODE OF OPERATION
BC40D_V_PU_ON_10P_SC1_3P3  Cell operated at 3.3(nom)
|BC40D_V_PU_ON_10P_SC1_3P3; BUFFER WITH WEAK_PULLUP_ON AT 10% SUPPLY
|VARIATION WITH SC1=1 MEANING SLOW MODE OF OPERATION
|   BC1833DV40DCPBFBP18LL_RXLL_SSDLH_135U
[Model Selector] bc1833dv40dcpbfbp18ll_rxll_ssdlh_135u
|SC1 IS A SLEW RATE CONTROL PIN
|5% SUPPLY VARIATION MODES WITH 1.8V NOM SUPPLY
BC40D_H_PUPDOFF_5P_SC1_1P8  Cell operated at 1.8(nom)
|BC40D_H_PUPDOFF_5P_SC1_1P8; BUFFER WITH WEAK PULUP/PULLDOWN OFF AT 5% SUPPLY
|VARIATION WITH SC1=1 MEANING SLOW MODE OF OPERATION
BC40D_H_PD_ON_5P_!SC1_1P8  Cell operated at 1.8(nom)
|BC40D_H_PD_ON_5P_!SC1_1P8; BUFFER WITH WEAK_PULLDOWN_ON AT 5% SUPPLY
|VARIATION WITH SC1=0 MEANING FAST MODE OF OPERATION
BC40D_H_PD_ON_5P_SC1_1P8  Cell operated at 1.8(nom)
|BC40D_H_PD_ON_5P_SC1_1P8; BUFFER WITH WEAK_PULLDOWN_ON AT 5% SUPPLY
|VARIATION WITH SC1=1 MEANING SLOW MODE OF OPERATION
BC40D_H_PU_ON_5P_!SC1_1P8  Cell operated at 1.8(nom)
|BC40D_H_PU_ON_5P_!SC1_1P8; BUFFER WITH WEAK_PULLUP_ON AT 5% SUPPLY
|VARIATION WITH SC1=0 MEANING FAST MODE OF OPERATION
BC40D_H_PUPDOFF_5P_!SC1_1P8  Cell operated at 1.8(nom)
|BC40D_H_PUPDOFF_5P_!SC1_1P8; BUFFER WITH WEAK PULUP/PULLDOWN OFF AT 5% SUPPLY
|VARIATION WITH SC1=0 MEANING FAST MODE OF OPERATION
BC40D_H_PU_ON_5P_SC1_1P8  Cell operated at 1.8(nom)
|BC40D_H_PU_ON_5P_SC1_1P8; BUFFER WITH WEAK_PULLUP_ON AT 5% SUPPLY
|VARIATION WITH SC1=1 MEANING SLOW MODE OF OPERATION
|5% SUPPLY VARIATION MODES WITH 3.3V NOM SUPPLY
BC40D_H_PUPDOFF_5P_SC1_3P3  Cell operated at 3.3(nom)
|BC40D_H_PUPDOFF_5P_SC1_3P3; BUFFER WITH WEAK PULUP/PULLDOWN OFF AT 5% SUPPLY
|VARIATION WITH SC1=1 MEANING SLOW MODE OF OPERATION
BC40D_H_PD_ON_5P_!SC1_3P3  Cell operated at 3.3(nom)
|BC40D_H_PD_ON_5P_!SC1_3P3; BUFFER WITH WEAK_PULLDOWN_ON AT 5% SUPPLY
|VARIATION WITH SC1=0 MEANING FAST MODE OF OPERATION
BC40D_H_PD_ON_5P_SC1_3P3  Cell operated at 3.3(nom)
|BC40D_H_PD_ON_5P_SC1_3P3; BUFFER WITH WEAK_PULLDOWN_ON AT 5% SUPPLY
|VARIATION WITH SC1=1 MEANING SLOW MODE OF OPERATION
BC40D_H_PU_ON_5P_!SC1_3P3  Cell operated at 3.3(nom)
|BC40D_H_PU_ON_5P_!SC1_3P3; BUFFER WITH WEAK_PULLUP_ON AT 5% SUPPLY
|VARIATION WITH SC1=0 MEANING FAST MODE OF OPERATION
BC40D_H_PUPDOFF_5P_!SC1_3P3  Cell operated at 3.3(nom)
|BC40D_H_PUPDOFF_5P_!SC1_3P3; BUFFER WITH WEAK PULUP/PULLDOWN OFF AT 5% SUPPLY
|VARIATION WITH SC1=0 MEANING FAST MODE OF OPERATION
BC40D_H_PU_ON_5P_SC1_3P3  Cell operated at 3.3(nom)
|BC40D_H_PU_ON_5P_SC1_3P3; BUFFER WITH WEAK_PULLUP_ON AT 5% SUPPLY
|VARIATION WITH SC1=1 MEANING SLOW MODE OF OPERATION
| 10% SUPPLY VARIATION MODES WITH 1.8V NOM SUPPLY
BC40D_H_PUPDOFF_10P_SC1_1P8  Cell operated at 1.8(nom)
|BC40D_H_PUPDOFF_10P_SC1_1P8; BUFFER WITH WEAK PULUP/PULLDOWN OFF AT 10% SUPPLY
|VARIATION WITH SC1=1 MEANING SLOW MODE OF OPERATION
BC40D_H_PD_ON_10P_!SC1_1P8  Cell operated at 1.8(nom)
|BC40D_H_PD_ON_10P_!SC1_1P8; BUFFER WITH WEAK_PULLDOWN_ON AT 10% SUPPLY
|VARIATION WITH SC1=0 MEANING FAST MODE OF OPERATION
BC40D_H_PD_ON_10P_SC1_1P8  Cell operated at 1.8(nom)
|BC40D_H_PD_ON_10P_SC1_1P8; BUFFER WITH WEAK_PULLDOWN_ON AT 10% SUPPLY
|VARIATION WITH SC1=1 MEANING SLOW MODE OF OPERATION
BC40D_H_PU_ON_10P_!SC1_1P8  Cell operated at 1.8(nom)
|BC40D_H_PU_ON_10P_!SC1_1P8; BUFFER WITH WEAK_PULLUP_ON AT 10% SUPPLY
|VARIATION WITH SC1=0 MEANING FAST MODE OF OPERATION
BC40D_H_PUPDOFF_10P_!SC1_1P8  Cell operated at 1.8(nom)
|BC40D_H_PUPDOFF_10P_!SC1_1P8; BUFFER WITH WEAK PULUP/PULLDOWN OFF AT 10% SUPPLY
|VARIATION WITH SC1=0 MEANING FAST MODE OF OPERATION
BC40D_H_PU_ON_10P_SC1_1P8  Cell operated at 1.8(nom)
|BC40D_H_PU_ON_10P_SC1_1P8; BUFFER WITH WEAK_PULLUP_ON AT 10% SUPPLY
|VARIATION WITH SC1=1 MEANING SLOW MODE OF OPERATION
| 10% SUPPLY VARIATION MODES WITH 3.3V NOM SUPPLY
BC40D_H_PUPDOFF_10P_SC1_3P3  Cell operated at 3.3(nom)
|BC40D_H_PUPDOFF_10P_SC1_3P3; BUFFER WITH WEAK PULUP/PULLDOWN OFF AT 10% SUPPLY
|VARIATION WITH SC1=1 MEANING SLOW MODE OF OPERATION
BC40D_H_PD_ON_10P_!SC1_3P3  Cell operated at 3.3(nom)
|BC40D_H_PD_ON_10P_!SC1_3P3; BUFFER WITH WEAK_PULLDOWN_ON 10% SUPPLY
|VARIATION WITH SC1=0 MEANING FAST MODE OF OPERATION
BC40D_H_PD_ON_10P_SC1_3P3  Cell operated at 3.3(nom)
|BC40D_H_PD_ON_10P_SC1_3P3; BUFFER WITH WEAK_PULLDOWN_ON AT 10% SUPPLY
|VARIATION WITH SC1=1 MEANING SLOW MODE OF OPERATION
BC40D_H_PU_ON_10P_!SC1_3P3  Cell operated at 3.3(nom)
|BC40D_H_PU_ON_10P_!SC1_3P3; BUFFER WITH WEAK_PULLUP_ON AT 10% SUPPLY
|VARIATION WITH SC1=0 MEANING FAST MODE OF OPERATION
BC40D_H_PUPDOFF_10P_!SC1_3P3  Cell operated at 3.3(nom)
|BC40D_H_PUPDOFF_10P_!SC1_3P3; BUFFER WITH WEAK PULUP/PULLDOWN OFF AT 10% SUPPLY
|VARIATION WITH SC1=0 MEANING FAST MODE OF OPERATION
BC40D_H_PU_ON_10P_SC1_3P3  Cell operated at 3.3(nom)
|BC40D_H_PU_ON_10P_SC1_3P3; BUFFER WITH WEAK_PULLUP_ON AT 10% SUPPLY
|VARIATION WITH SC1=1 MEANING SLOW MODE OF OPERATION
|   BC1833DV40DCPBFBP18LL_RXLL_SSDLV_135U
[Model Selector] bc1833dv40dcpbfbp18ll_rxll_ssdlv_135u
|SC1 IS A SLEW RATE CONTROL PIN
|5% SUPPLY VARIATION MODES WITH 1.8V NOM SUPPLY
BC40D_V_PUPDOFF_5P_SC1_1P8  Cell operated at 1.8(nom)
|BC40D_V_PUPDOFF_5P_SC1_1P8; BUFFER WITH WEAK PULUP/PULLDOWN OFF AT 5% SUPPLY
|VARIATION WITH SC1=1 MEANING SLOW MODE OF OPERATION
BC40D_V_PD_ON_5P_!SC1_1P8  Cell operated at 1.8(nom)
|BC40D_V_PD_ON_5P_!SC1_1P8; BUFFER WITH WEAK_PULLDOWN_ON AT 5% SUPPLY
|VARIATION WITH SC1=0 MEANING FAST MODE OF OPERATION
BC40D_V_PD_ON_5P_SC1_1P8  Cell operated at 1.8(nom)
|BC40D_V_PD_ON_5P_SC1_1P8; BUFFER WITH WEAK_PULLDOWN_ON AT 5% SUPPLY
|VARIATION WITH SC1=1 MEANING SLOW MODE OF OPERATION
BC40D_V_PU_ON_5P_!SC1_1P8  Cell operated at 1.8(nom)
|BC40D_V_PU_ON_5P_!SC1_1P8; BUFFER WITH WEAK_PULLUP_ON AT 5% SUPPLY
|VARIATION WITH SC1=0 MEANING FAST MODE OF OPERATION
BC40D_V_PUPDOFF_5P_!SC1_1P8  Cell operated at 1.8(nom)
|BC40D_V_PUPDOFF_5P_!SC1_1P8; BUFFER WITH WEAK PULUP/PULLDOWN OFF AT 5% SUPPLY
|VARIATION WITH SC1=0 MEANING FAST MODE OF OPERATION
BC40D_V_PU_ON_5P_SC1_1P8  Cell operated at 1.8(nom)
|BC40D_V_PU_ON_5P_SC1_1P8; BUFFER WITH WEAK_PULLUP_ON AT 5% SUPPLY
|VARIATION WITH SC1=1 MEANING SLOW MODE OF OPERATION
|5% SUPPLY VARIATION MODES WITH 3.3V NOM SUPPLY
BC40D_V_PUPDOFF_5P_SC1_3P3  Cell operated at 3.3(nom)
|BC40D_V_PUPDOFF_5P_SC1_3P3; BUFFER WITH WEAK PULUP/PULLDOWN OFF AT 5% SUPPLY
|VARIATION WITH SC1=1 MEANING SLOW MODE OF OPERATION
BC40D_V_PD_ON_5P_!SC1_3P3  Cell operated at 3.3(nom)
|BC40D_V_PD_ON_5P_!SC1_3P3; BUFFER WITH WEAK_PULLDOWN_ON AT 5% SUPPLY
|VARIATION WITH SC1=0 MEANING FAST MODE OF OPERATION
BC40D_V_PD_ON_5P_SC1_3P3  Cell operated at 3.3(nom)
|BC40D_V_PD_ON_5P_SC1_3P3; BUFFER WITH WEAK_PULLDOWN_ON AT 5% SUPPLY
|VARIATION WITH SC1=1 MEANING SLOW MODE OF OPERATION
BC40D_V_PU_ON_5P_!SC1_3P3  Cell operated at 3.3(nom)
|BC40D_V_PU_ON_5P_!SC1_3P3; BUFFER WITH WEAK_PULLUP_ON AT 5% SUPPLY
|VARIATION WITH SC1=0 MEANING FAST MODE OF OPERATION
BC40D_V_PUPDOFF_5P_!SC1_3P3  Cell operated at 3.3(nom)
|BC40D_V_PUPDOFF_5P_!SC1_3P3; BUFFER WITH WEAK PULUP/PULLDOWN OFF AT 5% SUPPLY
|VARIATION WITH SC1=0 MEANING FAST MODE OF OPERATION
BC40D_V_PU_ON_5P_SC1_3P3  Cell operated at 3.3(nom)
|BC40D_V_PU_ON_5P_SC1_3P3; BUFFER WITH WEAK_PULLUP_ON AT 5% SUPPLY
|VARIATION WITH SC1=1 MEANING SLOW MODE OF OPERATION
| 10% SUPPLY VARIATION MODES WITH 1.8V NOM SUPPLY
BC40D_V_PUPDOFF_10P_SC1_1P8  Cell operated at 1.8(nom)
|BC40D_V_PUPDOFF_10P_SC1_1P8; BUFFER WITH WEAK PULUP/PULLDOWN OFF AT 10% SUPPLY
|VARIATION WITH SC1=1 MEANING SLOW MODE OF OPERATION
BC40D_V_PD_ON_10P_!SC1_1P8  Cell operated at 1.8(nom)
|BC40D_V_PD_ON_10P_!SC1_1P8; BUFFER WITH WEAK_PULLDOWN_ON AT 10% SUPPLY
|VARIATION WITH SC1=0 MEANING FAST MODE OF OPERATION
BC40D_V_PD_ON_10P_SC1_1P8  Cell operated at 1.8(nom)
|BC40D_V_PD_ON_10P_SC1_1P8; BUFFER WITH WEAK_PULLDOWN_ON AT 10% SUPPLY
|VARIATION WITH SC1=1 MEANING SLOW MODE OF OPERATION
BC40D_V_PU_ON_10P_!SC1_1P8  Cell operated at 1.8(nom)
|BC40D_V_PU_ON_10P_!SC1_1P8; BUFFER WITH WEAK_PULLUP_ON AT 10% SUPPLY
|VARIATION WITH SC1=0 MEANING FAST MODE OF OPERATION
BC40D_V_PUPDOFF_10P_!SC1_1P8  Cell operated at 1.8(nom)
|BC40D_V_PUPDOFF_10P_!SC1_1P8; BUFFER WITH WEAK PULUP/PULLDOWN OFF AT 10% SUPPLY
|VARIATION WITH SC1=0 MEANING FAST MODE OF OPERATION
BC40D_V_PU_ON_10P_SC1_1P8  Cell operated at 1.8(nom)
|BC40D_V_PU_ON_10P_SC1_1P8; BUFFER WITH WEAK_PULLUP_ON AT 10% SUPPLY
|VARIATION WITH SC1=1 MEANING SLOW MODE OF OPERATION
| 10% SUPPLY VARIATION MODES WITH 3.3V NOM SUPPLY
BC40D_V_PUPDOFF_10P_SC1_3P3  Cell operated at 3.3(nom)
|BC40D_V_PUPDOFF_10P_SC1_3P3; BUFFER WITH WEAK PULUP/PULLDOWN OFF AT 10% SUPPLY
|VARIATION WITH SC1=1 MEANING SLOW MODE OF OPERATION
BC40D_V_PD_ON_10P_!SC1_3P3  Cell operated at 3.3(nom)
|BC40D_V_PD_ON_10P_!SC1_3P3; BUFFER WITH WEAK_PULLDOWN_ON 10% SUPPLY
|VARIATION WITH SC1=0 MEANING FAST MODE OF OPERATION
BC40D_V_PD_ON_10P_SC1_3P3  Cell operated at 3.3(nom)
|BC40D_V_PD_ON_10P_SC1_3P3; BUFFER WITH WEAK_PULLDOWN_ON AT 10% SUPPLY
|VARIATION WITH SC1=1 MEANING SLOW MODE OF OPERATION
BC40D_V_PU_ON_10P_!SC1_3P3  Cell operated at 3.3(nom)
|BC40D_V_PU_ON_10P_!SC1_3P3; BUFFER WITH WEAK_PULLUP_ON AT 10% SUPPLY
|VARIATION WITH SC1=0 MEANING FAST MODE OF OPERATION
BC40D_V_PUPDOFF_10P_!SC1_3P3  Cell operated at 3.3(nom)
|BC40D_V_PUPDOFF_10P_!SC1_3P3; BUFFER WITH WEAK PULUP/PULLDOWN OFF AT 10% SUPPLY
|VARIATION WITH SC1=0 MEANING FAST MODE OF OPERATION
BC40D_V_PU_ON_10P_SC1_3P3  Cell operated at 3.3(nom)
|BC40D_V_PU_ON_10P_SC1_3P3; BUFFER WITH WEAK_PULLUP_ON AT 10% SUPPLY
|VARIATION WITH SC1=1 MEANING SLOW MODE OF OPERATION
|   BC1833DV40DCPBFBP18LL_SSDLH_135U
[Model Selector] bc1833dv40dcpbfbp18ll_ssdlh_135u
|SC1 IS A SLEW RATE CONTROL PIN
|5% SUPPLY VARIATION MODES WITH 1.8V NOM SUPPLY
BC40D_H_PUPDOFF_5P_SC1_1P8  Cell operated at 1.8(nom)
|BC40D_H_PUPDOFF_5P_SC1_1P8; BUFFER WITH WEAK PULUP/PULLDOWN OFF AT 5% SUPPLY
|VARIATION WITH SC1=1 MEANING SLOW MODE OF OPERATION
BC40D_H_PD_ON_5P_!SC1_1P8  Cell operated at 1.8(nom)
|BC40D_H_PD_ON_5P_!SC1_1P8; BUFFER WITH WEAK_PULLDOWN_ON AT 5% SUPPLY
|VARIATION WITH SC1=0 MEANING FAST MODE OF OPERATION
BC40D_H_PD_ON_5P_SC1_1P8  Cell operated at 1.8(nom)
|BC40D_H_PD_ON_5P_SC1_1P8; BUFFER WITH WEAK_PULLDOWN_ON AT 5% SUPPLY
|VARIATION WITH SC1=1 MEANING SLOW MODE OF OPERATION
BC40D_H_PU_ON_5P_!SC1_1P8  Cell operated at 1.8(nom)
|BC40D_H_PU_ON_5P_!SC1_1P8; BUFFER WITH WEAK_PULLUP_ON AT 5% SUPPLY
|VARIATION WITH SC1=0 MEANING FAST MODE OF OPERATION
BC40D_H_PUPDOFF_5P_!SC1_1P8  Cell operated at 1.8(nom)
|BC40D_H_PUPDOFF_5P_!SC1_1P8; BUFFER WITH WEAK PULUP/PULLDOWN OFF AT 5% SUPPLY
|VARIATION WITH SC1=0 MEANING FAST MODE OF OPERATION
BC40D_H_PU_ON_5P_SC1_1P8  Cell operated at 1.8(nom)
|BC40D_H_PU_ON_5P_SC1_1P8; BUFFER WITH WEAK_PULLUP_ON AT 5% SUPPLY
|VARIATION WITH SC1=1 MEANING SLOW MODE OF OPERATION
|5% SUPPLY VARIATION MODES WITH 3.3V NOM SUPPLY
BC40D_H_PUPDOFF_5P_SC1_3P3  Cell operated at 3.3(nom)
|BC40D_H_PUPDOFF_5P_SC1_3P3; BUFFER WITH WEAK PULUP/PULLDOWN OFF AT 5% SUPPLY
|VARIATION WITH SC1=1 MEANING SLOW MODE OF OPERATION
BC40D_H_PD_ON_5P_!SC1_3P3  Cell operated at 3.3(nom)
|BC40D_H_PD_ON_5P_!SC1_3P3; BUFFER WITH WEAK_PULLDOWN_ON AT 5% SUPPLY
|VARIATION WITH SC1=0 MEANING FAST MODE OF OPERATION
BC40D_H_PD_ON_5P_SC1_3P3  Cell operated at 3.3(nom)
|BC40D_H_PD_ON_5P_SC1_3P3; BUFFER WITH WEAK_PULLDOWN_ON AT 5% SUPPLY
|VARIATION WITH SC1=1 MEANING SLOW MODE OF OPERATION
BC40D_H_PU_ON_5P_!SC1_3P3  Cell operated at 3.3(nom)
|BC40D_H_PU_ON_5P_!SC1_3P3; BUFFER WITH WEAK_PULLUP_ON AT 5% SUPPLY
|VARIATION WITH SC1=0 MEANING FAST MODE OF OPERATION
BC40D_H_PUPDOFF_5P_!SC1_3P3  Cell operated at 3.3(nom)
|BC40D_H_PUPDOFF_5P_!SC1_3P3; BUFFER WITH WEAK PULUP/PULLDOWN OFF AT 5% SUPPLY
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| Models and submodels in the file (68): BC40D_H_PUPDOFF_5P_SC1_1P8 (I/O), BC40D_H_PD_ON_5P_!SC1_1P8 (I/O), BC40D_H_PD_ON_5P_SC1_1P8 (I/O), BC40D_H_PU_ON_5P_!SC1_1P8 (I/O), BC40D_H_PUPDOFF_5P_!SC1_1P8 (I/O), BC40D_H_PU_ON_5P_SC1_1P8 (I/O), BC40D_H_PUPDOFF_5P_SC1_3P3 (I/O), BC40D_H_PD_ON_5P_!SC1_3P3 (I/O), BC40D_H_PD_ON_5P_SC1_3P3 (I/O), BC40D_H_PU_ON_5P_!SC1_3P3 (I/O), BC40D_H_PUPDOFF_5P_!SC1_3P3 (I/O), BC40D_H_PU_ON_5P_SC1_3P3 (I/O), BC40D_H_PUPDOFF_10P_SC1_1P8 (I/O), BC40D_H_PD_ON_10P_!SC1_1P8 (I/O), BC40D_H_PD_ON_10P_SC1_1P8 (I/O), BC40D_H_PU_ON_10P_!SC1_1P8 (I/O), BC40D_H_PUPDOFF_10P_!SC1_1P8 (I/O), BC40D_H_PU_ON_10P_SC1_1P8 (I/O), BC40D_H_PUPDOFF_10P_SC1_3P3 (I/O), BC40D_H_PD_ON_10P_!SC1_3P3 (I/O), BC40D_H_PD_ON_10P_SC1_3P3 (I/O), BC40D_H_PU_ON_10P_!SC1_3P3 (I/O), BC40D_H_PUPDOFF_10P_!SC1_3P3 (I/O), BC40D_H_PU_ON_10P_SC1_3P3 (I/O), BC40D_V_PUPDOFF_5P_SC1_1P8 (I/O), BC40D_V_PD_ON_5P_!SC1_1P8 (I/O), BC40D_V_PD_ON_5P_SC1_1P8 (I/O), BC40D_V_PU_ON_5P_!SC1_1P8 (I/O), BC40D_V_PUPDOFF_5P_!SC1_1P8 (I/O), BC40D_V_PU_ON_5P_SC1_1P8 (I/O), BC40D_V_PUPDOFF_5P_SC1_3P3 (I/O), BC40D_V_PD_ON_5P_!SC1_3P3 (I/O), BC40D_V_PD_ON_5P_SC1_3P3 (I/O), BC40D_V_PU_ON_5P_!SC1_3P3 (I/O), BC40D_V_PUPDOFF_5P_!SC1_3P3 (I/O), BC40D_V_PU_ON_5P_SC1_3P3 (I/O), BC40D_V_PUPDOFF_10P_SC1_1P8 (I/O), BC40D_V_PD_ON_10P_!SC1_1P8 (I/O), BC40D_V_PD_ON_10P_SC1_1P8 (I/O), BC40D_V_PU_ON_10P_!SC1_1P8 (I/O), BC40D_V_PUPDOFF_10P_!SC1_1P8 (I/O), BC40D_V_PU_ON_10P_SC1_1P8 (I/O), BC40D_V_PUPDOFF_10P_SC1_3P3 (I/O), BC40D_V_PD_ON_10P_!SC1_3P3 (I/O), BC40D_V_PD_ON_10P_SC1_3P3 (I/O), BC40D_V_PU_ON_10P_!SC1_3P3 (I/O), BC40D_V_PUPDOFF_10P_!SC1_3P3 (I/O), BC40D_V_PU_ON_10P_SC1_3P3 (I/O), BI2C1833_NORAML_5P_1P8 (I/O_open_drain), BI2C1833_NORAML_5P_3P3 (I/O_open_drain), BI2C1833_NORAML_10P_1P8 (I/O_open_drain), BI2C1833_NORAML_10P_3P3 (I/O_open_drain), IHHV_NORAML_5P_1P8 (Input), IHHV_NORAML_5P_3P3 (Input), IHHV_NORAML_10P_1P8 (Input), IHHV_NORAML_10P_3P3 (Input), IQ_SSDHH_PD_ON_5P_1P8 (Input), IQ_SSDHH_PU_ON_5P_1P8 (Input), IQ_SSDHH_PUPDOFF_5P_1P8 (Input), IQ_SSDHH_PD_ON_5P_3P3 (Input), IQ_SSDHH_PU_ON_5P_3P3 (Input), IQ_SSDHH_PUPDOFF_5P_3P3 (Input), IQ_SSDHH_PD_ON_10P_1P8 (Input), IQ_SSDHH_PU_ON_10P_1P8 (Input), IQ_SSDHH_PUPDOFF_10P_1P8 (Input), IQ_SSDHH_PD_ON_10P_3P3 (Input), IQ_SSDHH_PU_ON_10P_3P3 (Input), IQ_SSDHH_PUPDOFF_10P_3P3 (Input)
